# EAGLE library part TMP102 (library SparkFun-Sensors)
I2C degC temp sensor
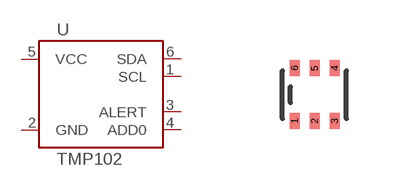
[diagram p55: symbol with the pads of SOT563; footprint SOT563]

Designator prefix U

## TMP102  [SOT563]
1  SCL
2  GND
3  ALERT
4  ADD0
5  VCC
6  SDA

## Footprint SOT563 (pad centres in mm)
smd 0.25 x 0.4: 1 -0.5,-0.66; 2 0,-0.66; 3 0.5,-0.66; 4 0.5,0.66; 5 0,0.66; 6 -0.5,0.67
